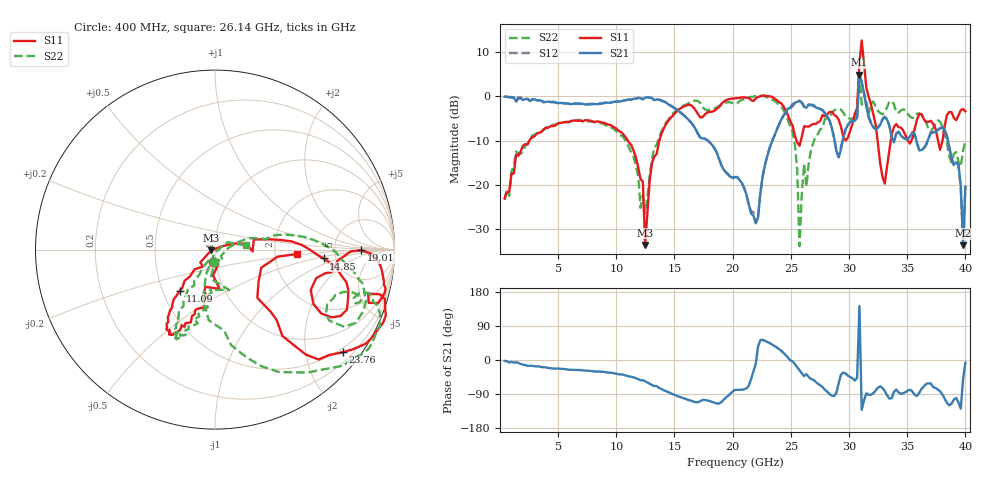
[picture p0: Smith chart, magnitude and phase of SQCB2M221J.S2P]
! Network Analyzer HP8722ES.07.66: Jul 25, 2000 Serial No. US39175408
! 27 Oct 2004  13:27:25
! Frequency  S11  S21  S12  S22
# HZ  S  DB R  50
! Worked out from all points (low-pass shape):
!   201 points, 400 MHz to 40 GHz, reference 50 ohm
!   highest |S21| = 4.90 dB at 30.89 GHz (marker M1); lowest = -33.7 dB at 39.8 GHz (marker M2)
!   |S21| within 3 dB of the highest: 30.83 GHz to 31.2 GHz (369.3 MHz wide, 1.19 % of centre)
!   lowest |S11| = -33.6 dB at 12.48 GHz (marker M3), VSWR 1.04, Z = 48 - j0.389 ohm
!   |S11| at or under -10 dB: start of sweep to 2.53 GHz; 11 GHz to 13.7 GHz (2.7 GHz wide, 21.9 % of centre); 32.46 GHz to 33.59 GHz (1.13 GHz wide, 3.42 % of centre)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
!   |S22| runs from -33.8 to 5.8 dB; largest |S21 - S12| = 0.27
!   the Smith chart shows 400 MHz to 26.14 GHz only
!   S11 on the Smith chart (normalised r, x): 400 MHz: 0.97, -0.14; 11.09 GHz: 0.61, -0.31; 14.85 GHz: 3.99, -0.63; 19.01 GHz: 9.74, -0.20; 23.76 GHz: 0.41, -2.78; 26.14 GHz: 2.69, -0.16
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4e8  -23.04 -97.7  -0.06 -2.3  -0.03 -1.7  -23.31 -93.5
7.132e9  -5.59 -118.6  -1.68 -27.6  -1.77 -28.3  -5.72 -114.3
1.1092e10  -10.41 -130.6  -0.68 -43.4  -0.68 -43.4  -11.52 -124.3
1.2478e10  -33.59 -168.8  -0.25 -55.8  -0.23 -56.1  -26.32 -45.1
1.3666e10  -10.28 11.0  -0.73 -73.5  -0.71 -73.2  -9.28 13.5
1.4854e10  -4.32 -4.7  -2.38 -90.2  -2.33 -90.5  -3.87 0.8
1.9012e10  -1.79 -0.2  -15.40 -111.3  -15.49 -110.7  -1.89 -17.3
2.02e10  -0.41 -9.9  -18.22 -78.9  -18.23 -78.5  -1.74 -19.3
2.3764e10  -0.80 -38.9  -7.66 33.9  -7.70 34.0  -1.32 -52.8
2.5348e10  -8.93 -48.7  -1.45 -11.0  -1.46 -11.5  -10.93 -103.4
2.5744e10  -11.16 -21.4  -1.01 -26.9  -0.94 -27.3  -33.85 -98.4
2.614e10  -6.76 -3.0  -2.39 -42.3  -2.27 -41.7  -15.24 7.7
2.6932e10  -6.21 -4.4  -1.90 -52.2  -2.21 -52.9  -10.45 30.5
2.911e10  -5.26 -89.4  -13.79 -61.3  -13.68 -60.2  -2.97 -33.5
3.0694e10  -2.62 70.8  -4.82 -47.2  -4.60 -47.3  -3.62 -110.0
3.0892e10  7.49 -27.6  4.90 142.7  5.31 134.6  5.83 -2.3
3.109e10  12.65 -67.0  3.25 -131.8  3.07 -131.9  -1.84 160.9
3.1486e10  2.03 -61.8  -2.19 -87.9  -2.13 -88.9  -1.31 -124.6
3.3466e10  -12.20 72.3  -6.71 -102.0  -6.53 -103.8  -1.23 -177.2
3.8218e10  -6.68 -50.2  -7.55 -102.1  -7.65 -104.8  -8.49 76.3
3.9802e10  -2.86 -121.4  -33.68 -49.9  -32.16 -35.6  -12.19 -106.6
4e10  -3.36 -135.4  -20.62 -6.9  -20.16 -7.3  -10.07 -114.0
